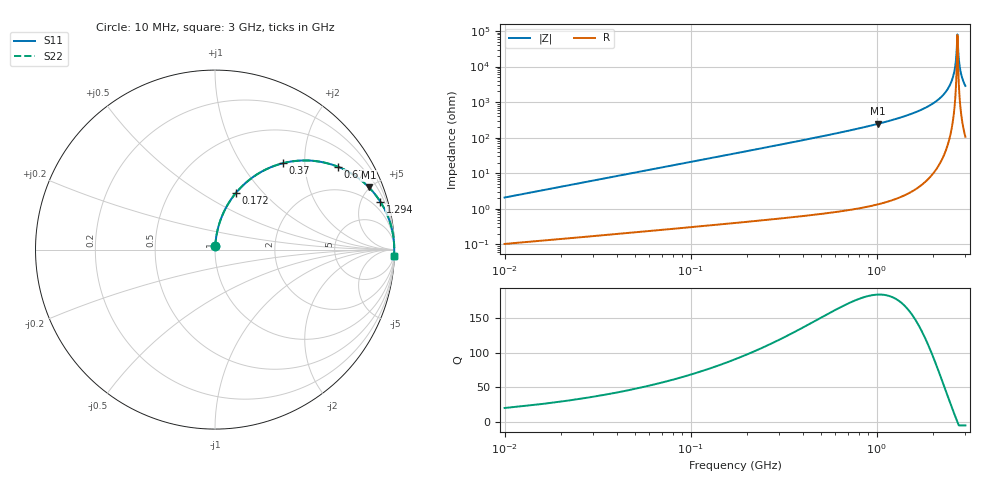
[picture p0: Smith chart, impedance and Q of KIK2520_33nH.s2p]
!version-2
!date-01.2022
!Series
# MHz S RI R 50
!Freq ReS11 ImS11 ReS21 ImS21 ReS12 ImS12 ReS22 ImS22
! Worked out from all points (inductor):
!   500 points, 10 MHz to 3 GHz, reference 50 ohm
!   read as one part in series: L = 33 nH near 22 MHz
!   highest Q = 184 at 1.018 GHz (marker M1), where L = 38.4 nH
!   self-resonance near 2.716 GHz
!   S11 on the Smith chart (normalised r, x): 10 MHz: 1.00, +0.04; 172 MHz: 1.01, +0.72; 370 MHz: 1.01, +1.56; 670 MHz: 1.02, +2.96; 1.294 GHz: 1.04, +6.94; 3 GHz: 3, -57
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10  0.00146 0.0207  0.9985 -0.0207  0.9985 -0.0207  0.00146 0.0207
34  0.00673 0.0699  0.9933 -0.0699  0.9933 -0.0699  0.00673 0.0699
64  0.0196 0.1298  0.9804 -0.1298  0.9804 -0.1298  0.0196 0.1298
172  0.1164 0.3152  0.8836 -0.3152  0.8836 -0.3152  0.1164 0.3152
370  0.3802 0.4816  0.6198 -0.4816  0.6198 -0.4816  0.3802 0.4816
514  0.5496 0.4943  0.4504 -0.4943  0.4504 -0.4943  0.5496 0.4943
670  0.6853 0.4614  0.3147 -0.4614  0.3147 -0.4614  0.6853 0.4614
1012  0.8544 0.35  0.1456 -0.35  0.1456 -0.35  0.8544 0.35
1018  0.8563 0.348  0.1437 -0.348  0.1437 -0.348  0.8563 0.348
1294  0.922 0.2653  0.078 -0.2653  0.078 -0.2653  0.922 0.2653
1510  0.9523 0.21  0.0477 -0.21  0.0477 -0.21  0.9523 0.21
2008  0.9871 0.1076  0.0129 -0.1076  0.0129 -0.1076  0.9871 0.1076
2308  0.9955 0.058  0.00452 -0.058  0.00452 -0.058  0.9955 0.058
2506  0.998 0.0288  0.00199 -0.0288  0.00199 -0.0288  0.998 0.0288
2644  0.9987 0.00984  0.00128 -0.00984  0.00128 -0.00984  0.9987 0.00984
2680  0.9988 0.00505  0.00122 -0.00505  0.00122 -0.00505  0.9988 0.00505
2716  0.9988 0.000328  0.00121 -0.000328  0.00121 -0.000328  0.9988 0.000328
2728  0.9988 -0.00123  0.00121 0.00123  0.00121 0.00123  0.9988 -0.00123
2764  0.9987 -0.00587  0.00125 0.00587  0.00125 0.00587  0.9987 -0.00587
2806  0.9986 -0.0112  0.00136 0.0112  0.00136 0.0112  0.9986 -0.0112
2884  0.9983 -0.0209  0.00169 0.0209  0.00169 0.0209  0.9983 -0.0209
3000  0.9975 -0.0349  0.00252 0.0349  0.00252 0.0349  0.9975 -0.0349
